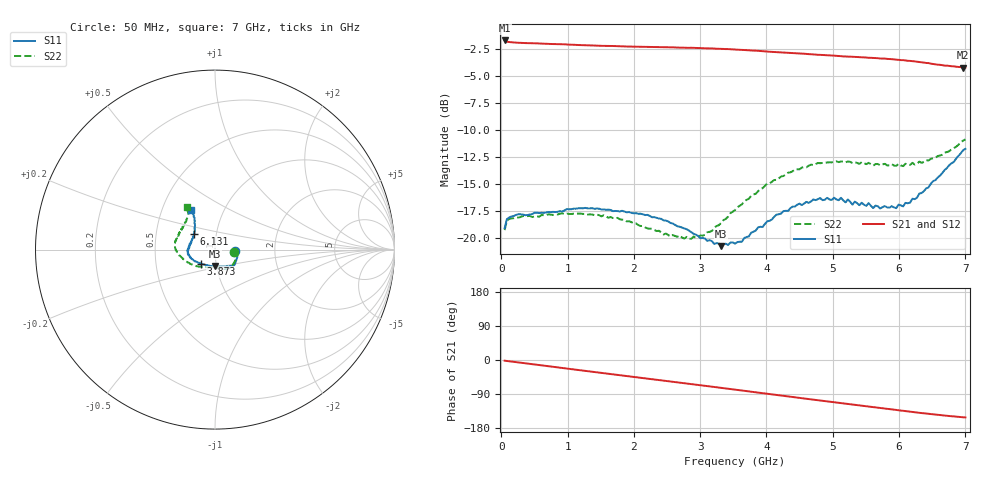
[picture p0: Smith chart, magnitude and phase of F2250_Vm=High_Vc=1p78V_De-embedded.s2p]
! Integrated Device Technology
! Corporate Headquarters
! 6024 Silver Creek Valley Road
! San Jose, CA 95138  USA
! Phone:  1-408-284-8200
! Toll Free:  1-800-223-1366
! Webpage:  http://www.idt.com/
! Timing and RF Division
! 515 Groton Road, Suite 102
! Westford, MA 01886-6024
! Device:  F2250
! Description: Voltage Variable RF Attenuator
! Frequency:  50.0 -  6000.00 MHz
! Package:  3x3 mm Thin QFN Plastic Package: 16 pin
! Ports:  2 RF, 3 DC
!  Pin  1  = GND
!  Pin  2  = NC
!  Pin  3  = RF1  = Port 1
!  Pin  4  = NC
!  Pin  5  = GND
!  Pin  6  = GND
!  Pin  7  = GND
!  Pin  8  = GND
!  Pin  9  = NC
!  Pin 10  = RF2  = Port 2
!  Pin 11  = NC
!  Pin 12  = GND
!  Pin 13  = GND
!  Pin 14  = VCNTRL
!  Pin 15  = VDD
!  Pin 16  = VMODE
! Vcntrl:  1.780 Volts
! Vmode:  +3.300 Volts
! Vdd:  +3.30  Volts
! Current:  1.324 mA
! Data:  The device was measured on a the F2250 evaluation board which has
!  individual transmission lines to the RF pins.  Data was collected
!  using a calibrated network analyzer.  The evaluation board was
!  de-embedded using a TRL calibration technique.
!  The reference plane is the edge of the package pin.
! Misc:  SN 10
!  Action Tracker AT0258
! Date Measured:  2014-11-26
! Date:  2015-10-15  MJV
! Note:
!  Integrated Device Technology supplies this data as a sample of measured
!  data at the package pin for this product.  Your particular data for this
!  product may vary.
!  Data was taken at 25 degrees C.
!  Integrated Device Technology reserves the right to change this data at anytime.
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# GHz S dB R 50
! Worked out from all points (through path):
!   201 points, 50 MHz to 7 GHz, reference 50 ohm
!   highest |S21| = -1.69 dB at 50 MHz (marker M1); lowest = -4.2 dB at 6.965 GHz (marker M2)
!   group delay of S21, straight-line fit = 60.9 ps
!   lowest |S11| = -20.7 dB at 3.317 GHz (marker M3), VSWR 1.20, Z = 48.9 - j9.07 ohm
!   |S11| at or under -10 dB: start of sweep to end of sweep
!   |S22| runs from -20.0 to -10.8 dB; largest |S21 - S12| = 0.0019
!   S11 on the Smith chart (normalised r, x): 50 MHz: 1.25, -0.02; 3.873 GHz: 0.84, -0.14; 6.131 GHz: 0.78, +0.14; 7 GHz: 0.70, +0.33
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0.05  -19.06 -4.7  -1.69 -1.9  -1.69 -1.9  -19.24 -6.2
0.08475  -18.23 -4.6  -1.80 -2.6  -1.79 -2.5  -18.37 -5.9
0.2585  -17.77 -10.7  -1.91 -6.4  -1.91 -6.4  -18.08 -13.2
1.2315  -17.22 -38.9  -2.12 -27.9  -2.12 -27.9  -17.74 -49.7
1.75275  -17.48 -45.8  -2.23 -39.0  -2.23 -39.1  -18.11 -60.9
2.37825  -18.17 -49.4  -2.32 -52.5  -2.32 -52.5  -19.30 -72.8
2.86475  -19.43 -61.3  -2.37 -63.3  -2.38 -63.4  -20.05 -94.8
3.07325  -20.02 -72.4  -2.42 -68.0  -2.42 -68.0  -19.67 -108.5
3.3165  -20.73 -91.6  -2.47 -73.6  -2.47 -73.6  -18.57 -124.9
3.525  -20.50 -108.6  -2.54 -78.3  -2.54 -78.3  -17.39 -136.7
3.8725  -18.99 -134.4  -2.65 -86.1  -2.67 -86.2  -15.64 -154.1
4.4285  -17.07 -159.2  -2.88 -98.4  -2.90 -98.5  -13.62 -173.5
4.7065  -16.40 -168.2  -2.98 -104.6  -2.99 -104.6  -13.22 179.8
5.1235  -16.25 -179.0  -3.15 -113.7  -3.14 -113.8  -12.89 169.8
5.29725  -16.89 175.6  -3.20 -117.4  -3.20 -117.5  -13.04 166.3
5.332  -16.60 174.1  -3.21 -118.3  -3.21 -118.3  -12.95 165.4
5.61  -17.20 166.5  -3.31 -124.3  -3.30 -124.3  -13.28 158.7
5.85325  -17.17 155.4  -3.41 -129.5  -3.42 -129.6  -13.26 151.5
6.13125  -16.76 142.9  -3.58 -135.5  -3.57 -135.6  -13.23 143.9
6.54825  -14.61 128.1  -3.89 -144.2  -3.89 -144.3  -12.56 130.3
6.96525  -11.85 121.1  -4.20 -151.1  -4.21 -151.2  -10.97 124.4
7  -11.72 120.7  -4.20 -151.6  -4.21 -151.7  -10.84 123.5
